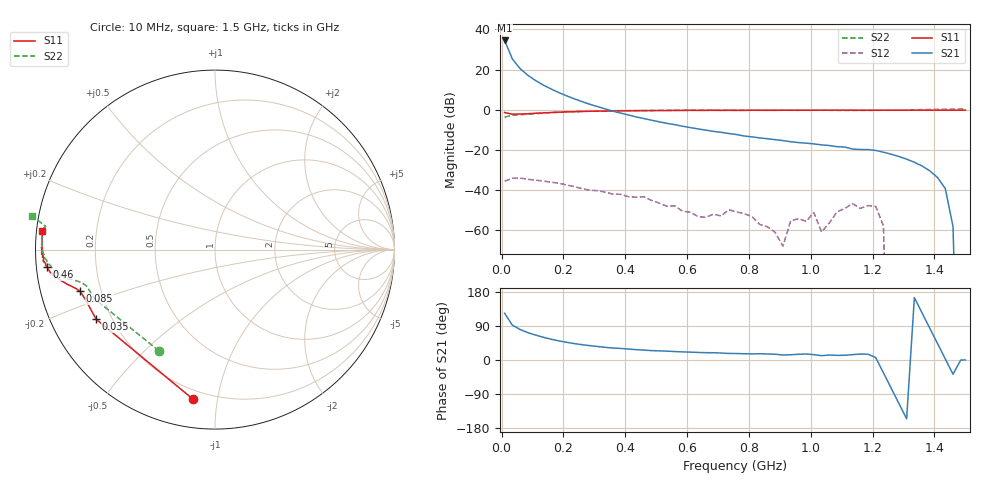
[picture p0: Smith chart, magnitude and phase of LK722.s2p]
! Date: Fri Jan 15 13:14:26 1999
!  POLYFET RF DEVICES
!  LP722/LK722
!  12.5Vdc		400ma
# MHZ  S  MA  R  50.0000
! SCATTERING PARAMETERS :
! Freq=MHz Mag[s11] Ang[s11] Mag[s21] Ang[s21] Mag[s12] Ang[s12] Mag[s22] Ang[s22]
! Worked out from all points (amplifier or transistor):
!   61 points, 10 MHz to 1.5 GHz, reference 50 ohm
!   highest |S21| = 34.5 dB at 10 MHz (marker M1)
!   |S21| within 3 dB of that: start of sweep to 18.15 MHz
!   S11 on the Smith chart (normalised r, x): 10 MHz: 0.15, -0.85; 35 MHz: 0.14, -0.27; 85 MHz: 0.12, -0.15; 460 MHz: 0.03, -0.05; 1.5 GHz: 0.02, +0.05
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10  0.8435 -98.3  53.08 123.3  0.01636 33.0  0.6452 -118.9
35  0.7674 -149.7  18.39 92.0  0.01925 3.3  0.7261 -158.0
60  0.7746 -159.3  10.56 80.6  0.01955 -8.0  0.7431 -164.1
85  0.787 -163.0  7.184 72.2  0.01819 -15.5  0.7677 -166.3
110  0.8085 -164.6  5.304 65.8  0.01726 -22.1  0.7924 -167.3
160  0.8444 -166.7  3.274 54.9  0.01536 -28.8  0.8385 -168.9
210  0.8752 -168.6  2.207 46.8  0.01309 -40.6  0.8697 -170.6
260  0.8962 -170.2  1.582 40.4  0.01062 -41.0  0.9017 -172.3
460  0.9434 -174.1  0.5975 26.1  0.00668 -57.5  0.949 -177.1
510  0.9475 -174.6  0.4947 24.2  0.00463 -56.9  0.9525 -178.3
760  0.9564 -177.4  0.2384 17.1  0.00279 -24.7  0.9558 177.6
910  0.9629 -178.9  0.1685 13.1  0.00039 -158.5  0.9661 175.0
935  0.9615 -178.7  0.1579 13.9  0.00166 81.4  0.9625 174.4
1010  0.9635 -178.8  0.1391 14.1  0.00268 91.2  0.9694 173.7
1035  0.9638 -179.7  0.1316 11.5  0.00088 83.5  0.9646 173.2
1135  0.964 179.7  0.1035 14.2  0.0045 77.7  0.9525 172.2
1210  0.9628 178.2  0.09579 6.5  0.00383 60.3  0.9573 172.0
1235  0.9632 177.9  0.08633 -33.9  0.00125 16.7  0.964 171.8
1260  0.9636 177.5  0.07687 -74.3  0 0.0  0.9707 171.6
1435  0.9665 174.8  0.01067 2.9  0 0.0  1.018 170.0
1485  0.9674 174.1  0 0.0  0 0.0  1.031 169.6
1500  0.9676 173.8  0 0.0  0 0.0  1.035 169.4
